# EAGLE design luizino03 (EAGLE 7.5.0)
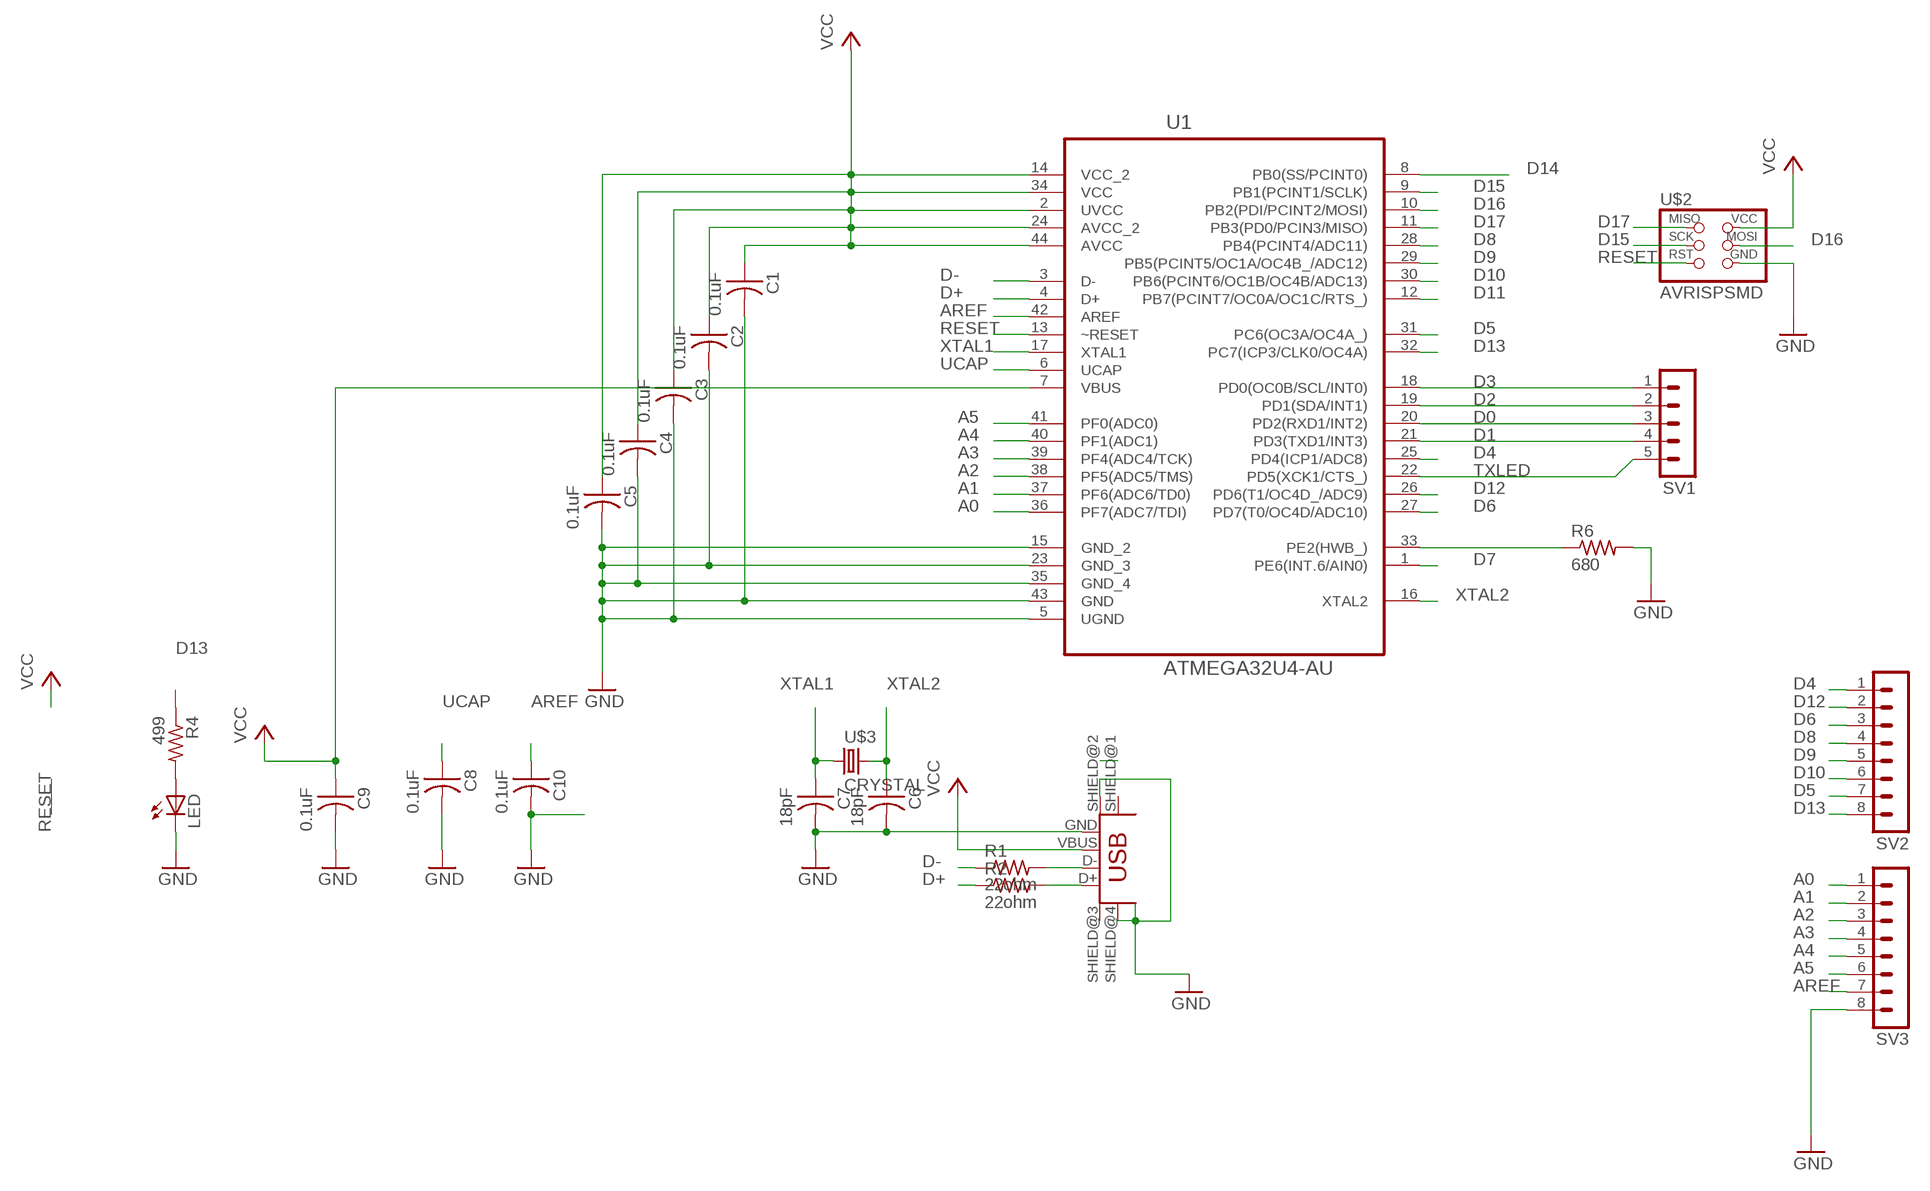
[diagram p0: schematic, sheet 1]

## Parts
C1  0.1uF  CAP-US1206FAB  [C1206FAB]
C2  0.1uF  CAP-US1206FAB  [C1206FAB]
C3  0.1uF  CAP-US1206FAB  [C1206FAB]
C4  0.1uF  CAP-US1206FAB  [C1206FAB]
C5  0.1uF  CAP-US1206FAB  [C1206FAB]
C6  18pF  CAP-US1206FAB  [C1206FAB]
C7  18pF  CAP-US1206FAB  [C1206FAB]
C8  0.1uF  CAP-US1206FAB  [C1206FAB]
C9  0.1uF  CAP-US1206FAB  [C1206FAB]
C10  0.1uF  CAP-US1206FAB  [C1206FAB]
LED  LED1206  [1206]
R1  22ohm  RES-US1206FAB  [R1206FAB]
R2  22ohm  RES-US1206FAB  [R1206FAB]
R4  499  RESISTOR1206  [1206]
R6  680  RES-US1206FAB  [R1206FAB]
SV1  MA05-1  [MA05-1]
SV2  MA08-1  [MA08-1]
SV3  MA08-1  [MA08-1]
U1  ATMEGA32U4-AU  [QFP80P1200X1200X120-44N]
U$1  USB_MINIB  [USB_MINIB]
U$2  AVRISPSMD  [2X03SMD]
U$3  CRYSTAL  [2-SMD-5X3MM]

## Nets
A0: SV3.1 U1.36(PF7(ADC7/TDI))
A1: SV3.2 U1.37(PF6(ADC6/TD0))
A2: SV3.3 U1.38(PF5(ADC5/TMS))
A3: SV3.4 U1.39(PF4(ADC4/TCK))
A4: SV3.5 U1.40(PF1(ADC1))
A5: SV3.6 U1.41(PF0(ADC0))
AREF: C10.1 SV3.7 U1.42(AREF)
D0: SV1.3 U1.20(PD2(RXD1/INT2))
D1: SV1.4 U1.21(PD3(TXD1/INT3))
D2: SV1.2 U1.19(PD1(SDA/INT1))
D3: SV1.1 U1.18(PD0(OC0B/SCL/INT0))
D4: SV2.1 U1.25(PD4(ICP1/ADC8))
D5: SV2.7 U1.31(PC6(OC3A/OC4A_))
D6: SV2.3 U1.27(PD7(T0/OC4D/ADC10))
D7: U1.1(PE6(INT.6/AIN0))
D8: SV2.4 U1.28(PB4(PCINT4/ADC11))
D9: SV2.5 U1.29(PB5(PCINT5/OC1A/OC4B_/ADC12))
D10: SV2.6 U1.30(PB6(PCINT6/OC1B/OC4B/ADC13))
D11: U1.12(PB7(PCINT7/OC0A/OC1C/RTS_))
D12: SV2.2 U1.26(PD6(T1/OC4D_/ADC9))
D13: R4.1 SV2.8 U1.32(PC7(ICP3/CLK0/OC4A))
D14: U1.8(PB0(SS/PCINT0))
D15: U1.9(PB1(PCINT1/SCLK)) U$2.3(SCK)
D16: U1.10(PB2(PDI/PCINT2/MOSI)) U$2.4(MOSI)
D17: U1.11(PB3(PD0/PCIN3/MISO)) U$2.1(MISO)
D+: R2.1 U1.4(D+)
D-: R1.1 U1.3(D-)
GND: C1.2 C2.2 C3.2 C4.2 C5.2 C6.2 C7.2 C8.2 C9.2 C10.2 LED.2(C) R6.2 SV3.8 U1.5(UGND) U1.15(GND_2) U1.23(GND_3) U1.35(GND_4) U1.43(GND) U$1.GND U$1.SHIELD@2(SHIELD1) U$1.SHIELD@4(SHIELD3) U$2.6(GND)
N$1: R1.2 U$1.D-
N$2: R2.2 U$1.D+
N$3: LED.1(A) R4.2
N$35: R6.1 U1.33(PE2(HWB_))
RESET: U1.13(~RESET) U$2.5(RST)
TXLED: SV1.5 U1.22(PD5(XCK1/CTS_))
UCAP: C8.1 U1.6(UCAP)
VCC: C1.1 C2.1 C3.1 C4.1 C5.1 C9.1 U1.2(UVCC) U1.7(VBUS) U1.14(VCC_2) U1.24(AVCC_2) U1.34(VCC) U1.44(AVCC) U$1.VBUS U$2.2(VCC)
XTAL1: C7.1 U1.17(XTAL1) U$3.P$1
XTAL2: C6.1 U1.16(XTAL2) U$3.P$2
Unconnected: U$1.SHIELD@1(SHIELD) U$1.SHIELD@3(SHIELD2)

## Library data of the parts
C1-C10 = fab:CAP-US
LED = ng:LED
R1 R2 R6 = fab:RES-US: Resistor (US Symbol)
R4 = ng:RESISTOR
SV1 = con-lstb:MA05-1: PIN HEADER; OC_FARNELL: unknown; OC_NEWARK: unknown
SV2 SV3 = con-lstb:MA08-1: PIN HEADER
U1 = Atmel_By_element14_Batch_1:ATMEGA32U4-AU: 8-bit Microcontroller with ISP Flash and USB Controller; MPN: ATMEGA32U4-AU; OC_FARNELL: 1748525; OC_NEWARK: 26R5633; PACKAGE: TQFP-44; SUPPLIER: Atmel
U$1 = fab:USB_MINIB
U$2 = fab:AVRISP
U$3 = fab:CRYSTAL

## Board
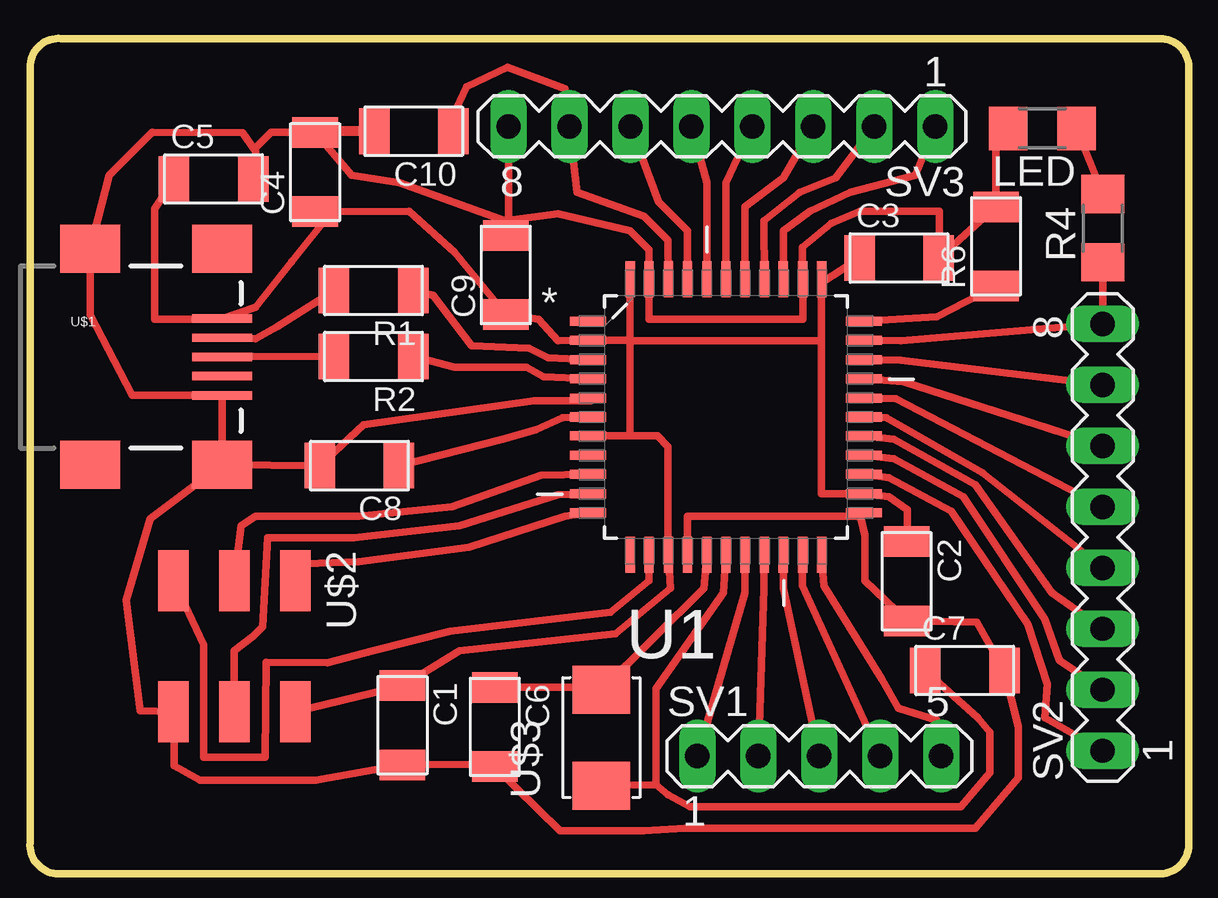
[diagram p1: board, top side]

No outline drawn. Coordinates in mm, seen from the top.
Copper layers (1*16): Top 0.035mm / dielectric 1.5mm / Bottom 0.035mm
Design rules "default *": minimum track width 10mil, minimum drill 24mil, track to track 0.4mm, track to pad 0.4mm, pad to pad 0.4mm, via to via 0.4mm, smd to smd 0.4mm, copper to edge 40mil, drill to drill 0.4mm, minimum pad ring 10mil, minimum via ring 8mil, stop-mask expansion 4mil, vias tented up to drill 0mil, thermal gap 10mil
Milling: 8 lines

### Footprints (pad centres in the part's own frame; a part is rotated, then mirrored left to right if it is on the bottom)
C1206FAB = smd 1.27 x 1.905: 1 -1.651,0; 2 1.651,0
1206 = smd 1.6 x 1.803: 1 -1.422,0; 2 1.422,0
R1206FAB = smd 1.27 x 1.905: 1 -1.651,0; 2 1.651,0
MA05-1 = drill 1.016 long: 1 -5.08,0; 2 -2.54,0; 3 0,0; 4 2.54,0; 5 5.08,0
MA08-1 = drill 1.016 long: 1 -8.89,0; 2 -6.35,0; 3 -3.81,0; 4 -1.27,0; 5 1.27,0; 6 3.81,0; 7 6.35,0; 8 8.89,0
QFP80P1200X1200X120-44N = smd 1.5 x 0.38: 1 -5.74,3.988; 2 -5.74,3.2; 3 -5.74,2.388; 4 -5.74,1.6; 5 -5.74,0.787; 6 -5.74,0; 7 -5.74,-0.787; 8 -5.74,-1.6; 9 -5.74,-2.388; 10 -5.74,-3.2; 11 -5.74,-3.988; 23 5.74,-3.988; 24 5.74,-3.2; 25 5.74,-2.388; 26 5.74,-1.6; 27 5.74,-0.787; 28 5.74,0; 29 5.74,0.787; 30 5.74,1.6; 31 5.74,2.388; 32 5.74,3.2; 33 5.74,3.988 | smd 0.38 x 1.5: 12 -3.988,-5.74; 13 -3.2,-5.74; 14 -2.388,-5.74; 15 -1.6,-5.74; 16 -0.787,-5.74; 17 0,-5.74; 18 0.787,-5.74; 19 1.6,-5.74; 20 2.388,-5.74; 21 3.2,-5.74; 22 3.988,-5.74; 34 3.988,5.74; 35 3.2,5.74; 36 2.388,5.74; 37 1.6,5.74; 38 0.787,5.74; 39 0,5.74; 40 -0.787,5.74; 41 -1.6,5.74; 42 -2.388,5.74; 43 -3.2,5.74; 44 -3.988,5.74
USB_MINIB = smd 2.5 x 0.35: D+ 3.77,0; D- 3.77,0.8; GND 3.77,-1.6; ID 3.77,-0.8; VBUS 3.77,1.6 | smd 2.5 x 2: SHIELD@1 -1.73,-4.5; SHIELD@2 -1.73,4.5; SHIELD@3 3.77,4.5; SHIELD@4 3.77,-4.5
2X03SMD = smd 2.54 x 1.27: 1 -2.54,2.54; 2 2.92,2.54; 3 -2.54,0; 4 2.92,0; 5 -2.54,-2.54; 6 2.92,-2.54
2-SMD-5X3MM = smd 2 x 2.4: P$1 -2,0; P$2 2,0

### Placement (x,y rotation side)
C1  40.23,5.39 270 top
C2  61.24,11.39 270 top
C3  60.93,24.85 0 top
C4  36.59,28.43 90 top
C5  32.35,28.14 0 top
C6  44.07,5.32 270 top
C7  63.67,7.66 0 top
C8  38.43,16.2 180 top
C9  44.54,24.15 90 top
C10  40.7,30.13 180 top
LED  66.9,30.25 180 top
R1  39.02,23.5 180 top
R2  39.02,20.75 180 top
R4  69.42,26.1 90 top
R6  64.97,25.34 90 top
SV1  57.6,4.1 0 top
SV2  69.42,13.21 90 top
SV3  53.54,30.34 180 top
U1  53.71,18.23 0 top
U$1  28.93,20.73 0 top
U$2  33.22,8.87 270 top
U$3  48.52,4.87 90 top

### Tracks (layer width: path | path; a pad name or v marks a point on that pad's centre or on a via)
A0
  Top 0.305: U1.36 56.1,26 57.2,26.8 58.9,27.6 61.6,28.3 SV3.1
A1
  Top 0.305: U1.37 55.3,26.4 56.8,27.6 58.3,28.2 SV3.2
A2
  Top 0.305: U1.38 54.5,27 56.1,28.2 SV3.3
A3
  Top 0.305: U1.39 53.7,28 SV3.4
A4
  Top 0.305: U1.40 52.93,27.99 SV3.5
A5
  Top 0.305: U1.41 52.1,26 50.9,27.2 SV3.6
AREF
  Top 0.305: 47,31.9 SV3.7 | U1.42 51.3,25.6 50.3,26.6 47.5,27.6 47,31.9 | 47,31.9 44.6,32.8 42.9,32 42.3,30.7 42.1,29.89 C10.1
D0
  Top 0.305: SV1.3 56.1,11.1 U1.20
D1
  Top 0.305: SV1.4 56.9,11.2 U1.21
D2
  Top 0.305: SV1.2 55.3,11.1 U1.19
D3
  Top 0.305: SV1.1 54.5,10.9 U1.18
D4
  Top 0.305: U1.25 60.5,15.7 63.1,14.3 66.3,9.6 67.1,7.1 67,5.7 SV2.1
D5
  Top 0.305: U1.31 61,20.6 SV2.7
D6
  Top 0.305: U1.27 60.7,17.3 64.1,15.4 67.3,10.9 SV2.3
D8
  Top 0.305: U1.28 60.4,18.2 64.4,15.9 SV2.4
D9
  Top 0.305: U1.29 60.8,19 SV2.5
D10
  Top 0.305: U1.30 61.1,19.7 SV2.6
D12
  Top 0.305: U1.26 60.7,16.5 63.6,14.9 67,9.8 67.6,8.1 SV2.2
D13
  Top 0.305: U1.32 61,21.4 SV2.8 R4.1
D15
  Top 0.305: U1.9 46,15.8 42.3,14.5 38.4,14.1 34.1,14.1 33.5,13.7 U$2.3
D16
  Top 0.305: U$2.4 33.2,8.5 34,9.1 34.4,9.5 34.6,13.2 38.2,13.2 42.6,13.7 46.7,15 U1.10
D17
  Top 0.305: U1.11 47,14.1 43,12.8 38.4,12.2 35.6,12.1 U$2.1
D+
  Top 0.305: U1.4 46.1,19.9 45.4,20.3 42.4,20.3 R2.1
D-
  Top 0.305: U1.3 46.3,20.7 45.5,21.1 43.1,21.2 41.5,23.3 R1.1
GND
  Top 0.305: U1.5 48.09,18.9 45.7,18.9 38.6,17.9 C8.2 U$1.SHIELD@4 | U1.15 52.1,14.1 59.31,14.1 | U1.23 59.31,14.1 | C5.2 34.1,28.24 34.1,29.3 34.04,29.38 | 44.5,26.4 46.7,26.7 49.7,26 50.5,25.2 U1.43 50.5,22.3 56.9,22.3 56.91,22.31 U1.35 56.9,25.3 58.1,26.3 59.3,26.8 62.6,26.8 C3.2 R6.2 64.96,30.18 LED.2 | 44.5,26.4 40.1,28 38.1,28.3 C4.2 34.75,30.09 34.04,29.38 | 59.31,14.1 59.5,13.3 59.5,11.4 C2.2 64.17,9.68 C7.2 65.9,5.3 65.9,3.2 64.1,1.1 52,1.1 50.3,1 46.8,1 C6.2 43.5,3.76 C1.2 36.6,3.1 31.8,3.1 30.7,3.7 U$2.6 29.3,6 28.7,10.6 29.7,14 U$1.SHIELD@4 | U$1.SHIELD@4 U$1.GND 28.97,19.13 27.2,22.5 U$1.SHIELD@2 28,28.3 29.8,30.1 33.56,30.07 34.04,29.38 | 44.5,26.4 C9.2 44.65,25.91 SV3.8
  Top 0.406: C10.2 36.59,30.13 C4.2
N$1
  Top 0.305: R1.2 35,22 34.1,21.5 U$1.D-
N$2
  Top 0.305: R2.2 U$1.D+
N$3
  Top 0.305: LED.1 R4.2
N$35
  Top 0.305: U1.33 62.5,22.4 R6.1
RESET
  Top 0.305: U1.13 50.5,11.4 48.9,10.1 42.2,9.3 39,8.5 37.1,8 34.53,8.02 34.51,4.05 31.94,4.05 31.94,8.74 U$2.5
TXLED
  Top 0.305: SV1.5 62.5,5.6 60.9,6.1 60.2,7.3 57.8,11.2 U1.22
UCAP
  Top 0.305: U1.6 46.9,18.2 45.8,17.7 44.4,17.3 C8.1
VCC
  Top 0.305: C3.1 57.79,23.88 U1.34 57.7,21.4 | 49.7,17.44 50.86,17.44 51.3,17 51.3,12.51 U1.14 51.4,11.1 49.1,9.2 42.6,8.5 C1.1 U$2.2 | 49.7,17.44 U1.7 | 57.7,21.4 49.7,21.4 | 49.7,21.43 49.7,23.97 U1.44 | U1.2 47.97,21.4 | 57.7,21.4 57.7,15.03 U1.24 60.5,14.9 61.27,14.36 C2.1 | 49.7,21.4 49.7,17.44 | 49.7,21.4 49.7,21.43 | 49.7,21.43 U1.2 | C5.1 29.9,26.9 29.9,22.3 32.7,22.3 U$1.VBUS 34.1,22.8 35.6,24.7 37.3,26.8 C4.1 40.5,26.8 42.4,25.1 C9.1 45.9,22.3 46.7,21.4 U1.2
XTAL1
  Top 0.305: C7.1 64.2,5.7 64.7,5.1 64.7,3.4 63.5,2 52.2,2 51.3,2.5 50.8,2.9 | 50.8,2.9 U$3.P$1 | 50.8,2.9 50.8,6.9 53.6,10.9 U1.17
XTAL2
  Top 0.305: U1.16 52.8,11.1 U$3.P$2 48.07,6.97 C6.1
